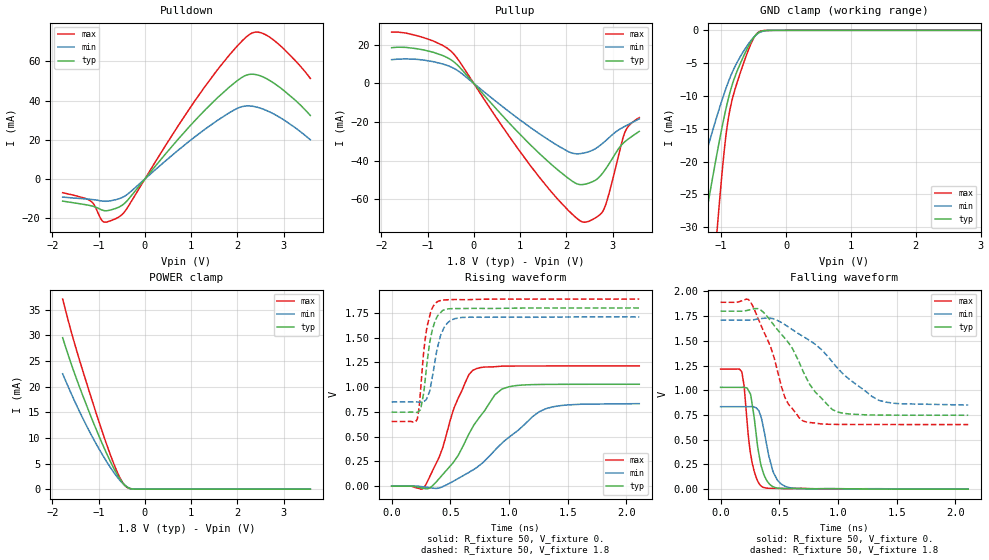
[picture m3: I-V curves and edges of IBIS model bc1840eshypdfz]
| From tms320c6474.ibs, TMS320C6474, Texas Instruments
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|   MODEL bc1840eshypdfz
[Model] bc1840eshypdfz
Model_type I/O
|C_comp_off 861.284f 847.135f 858.339f
|C_comp_on 527.297f 518.909f 520.66f
C_comp 694.29f 683.022f 689.5f
|Rth_i 17.068Meg 5.207Meg 37.052Meg
|Rth_r 37.693 52.451 28.255
|Rth_f 35.826 49.423 26.843
Vinl = 0.630
Vinh = 1.170
Vmeas = 0.9
Cref = 5pF
[Model Spec]
||   Typ   Min   Max
S_overshoot_high   2.100   2.010   2.190
Vinh   1.170   1.111   1.229
Vmeas   0.900   0.855   0.945
Vinl   0.630   0.599   0.662
S_overshoot_low   -0.300  -0.300  -0.300
[Receiver Thresholds]
Vth   = 0.900V
Vth_min = 0.855V
Vth_max = 0.945V
Vinh_ac = +270mV   || Undefined so set to Vinh_dc level
Vinh_dc = +270mV
Vinl_dc = -270mV
Vinl_ac = -270mV   || Undefined so set to Vinl_dc level
Tslew_ac = 5.0ns   || Undefined in specification - set to large value
|| Pointer to HSPICE models:
|ff ti_bc1840eshypdfz.mod ti_bc1840eshypdfz_ff
|tt ti_bc1840eshypdfz.mod ti_bc1840eshypdfz_tt
|ss ti_bc1840eshypdfz.mod ti_bc1840eshypdfz_ss
|| Spice2IBIS controls:
|View_IV No
[Temperature Range]  25   105   -40
|corevdd   1.100  1.045  1.155
[Voltage Range]   1.8   1.71   1.89
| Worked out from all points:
|   slope of the pulldown table from 0 to 0.27 V, typ, clamps not added: 34.7 ohm
|   slope of the pullup table from 0 to 0.27 V, typ, clamps not added: 36.5 ohm
|   GND clamp passes 1 mA (typ) near -0.49 V on its own axis
|   POWER clamp passes 1 mA (typ) near -0.46 V on its own axis
|   rising waveform, R_fixture 50, V_fixture 0.: 20-80 % time 324ps typ, 473ps min, 216ps max; typ from 0 V to 1.03 V
|   rising waveform, R_fixture 50, V_fixture 1.8: 20-80 % time 74.1ps typ, 88.5ps min, 65.9ps max; typ from 0.747 V to 1.8 V
|   falling waveform, R_fixture 50, V_fixture 0.: 20-80 % time 79.8ps typ, 93.5ps min, 67.9ps max; typ from 1.03 V to 0 V
|   falling waveform, R_fixture 50, V_fixture 1.8: 20-80 % time 326ps typ, 487ps min, 211ps max; typ from 1.8 V to 0.748 V
[Pulldown]
-1.779V   -11.3mA    -9.255mA   -7.029mA
-1.172V   -13.64mA   -10.42mA   -11.28mA
-885.2mV  -16.14mA   -11.37mA   -21.98mA
-500.8mV  -13.54mA   -9.552mA   -18.3mA
712mV     20.11mA    14.53mA    26.88mA
1.308V    35.38mA    25.54mA    47.47mA
1.973V    49.72mA    35.76mA    67.24mA
2.309V    53.44mA    37.14mA    74.38mA
2.531V    52.27mA    35.84mA    74.42mA
2.807V    48.57mA    32.88mA    70.44mA
3.257V    40.06mA    26.03mA    60.25mA
3.576V    32.4mA     20.01mA    51.29mA
[Pullup]
-1.776V   18.46mA    12.27mA    26.51mA
-1.094V   17.34mA    12.09mA    23.74mA
-449.6mV  11.48mA    8.028mA    15.63mA
1.218V    -31.64mA   -22.7mA    -42.35mA
2.035V    -48.96mA   -35.19mA   -65.49mA
2.339V    -52.35mA   -36.21mA   -71.56mA
2.62V     -50.22mA   -33.91mA   -69.7mA
2.799V    -46.01mA   -30.75mA   -65.79mA
2.907V    -42.28mA   -28.47mA   -58.43mA
3.264V    -30.24mA   -22.25mA   -25.49mA
3.384V    -28.03mA   -20.76mA   -21.13mA
3.579V    -24.83mA   -18.32mA   -17.71mA
[GND Clamp]
-1.779V   -59.56mA   -37.99mA   -119.5mA
-1.529V   -45.23mA   -29.11mA   -89.37mA
-1.387V   -37mA      -24.1mA    -71.41mA
-1.191V   -25.75mA   -17.29mA   -46.39mA
-1.053V   -18.18mA   -12.7mA    -29.3mA
-937.4mV  -12.45mA   -9.168mA   -16.96mA
-897.4mV  -10.73mA   -8.067mA   -13.92mA
-848.4mV  -8.901mA   -6.841mA   -11.32mA
-581.4mV  -2.472mA   -2.093mA   -3.018mA
-492.4mV  -1.021mA   -996.9uA   -1.09mA
-412.3mV  -275.8uA   -354.1uA   -211.8uA
3.576V    0A         0A         0A
[Power Clamp]
-1.779V   29.56mA    22.51mA    37.1mA
-1.614V   24.99mA    19.08mA    31.43mA
-1.455V   20.94mA    15.94mA    26.43mA
-1.164V   14.12mA    10.66mA    17.94mA
-930.5mV  9.056mA    6.904mA    11.45mA
-739.7mV  5.286mA    4.151mA    6.541mA
-601.9mV  2.905mA    2.406mA    3.416mA
-490.6mV  1.362mA    1.232mA    1.427mA
-400.5mV  513.7uA    525.3uA    451uA
-321mV    131.2uA    160.6uA    101.3uA
-225.5mV  9.942uA    19.46uA    5.634uA
3.579V    0A         0A         0A
[Ramp]
dV/dt_r .618/324.071p .501/473.431p .729/215.934p
dV/dt_f .632/326.322p .516/488.075p .742/210.701p
[Rising Waveform]
R_fixture = 50
V_fixture = 0.
0s        0V         1.05uV     0V
270ps     -21.74mV   -7.257mV   -23.39mV
325ps     -19.33mV   -14.8mV    96.12mV
405ps     75.94mV    -17.84mV   293.2mV
525ps     238.2mV    48.99mV    764.2mV
655ps     518.9mV    136.6mV    1.118V
720ps     649.3mV    183.5mV    1.186V
940ps     980.6mV    433.6mV    1.212V
1.32ns    1.028V     784.7mV    1.214V
2.11ns    1.029V     833.3mV    1.214V
[Rising Waveform]
R_fixture = 50
V_fixture = 1.8
V_fixture_min = 1.71
V_fixture_max = 1.89
0s        747.2mV    850.2mV    653.1mV
215ps     744.7mV    850.2mV    669.4mV
235ps     760.4mV    849.5mV    797.8mV
250ps     791.7mV    849.9mV    1.019V
300ps     1.23V      887.2mV    1.597V
345ps     1.57V      1.092V     1.795V
400ps     1.731V     1.443V     1.869V
475ps     1.789V     1.648V     1.883V
595ps     1.794V     1.704V     1.884V
2.11ns    1.8V       1.71V      1.89V
[Falling Waveform]
R_fixture = 50
V_fixture = 0.
0s        1.03V      834.2mV    1.215V
180ps     1.03V      834.2mV    1.187V
200ps     1.03V      834.2mV    1.047V
230ps     1.015V     834.2mV    626mV
270ps     852.2mV    834.1mV    260.6mV
320ps     399mV      801mV      73.28mV
365ps     162.1mV    622.5mV    17.59mV
450ps     23.32mV    168.4mV    8.658mV
580ps     6.889mV    17.31mV    5.07mV
2.11ns    375.6uV    685.6uV    140.3uV
[Falling Waveform]
R_fixture = 50
V_fixture = 1.8
V_fixture_min = 1.71
V_fixture_max = 1.89
0s        1.8V       1.71V      1.89V
255ps     1.816V     1.71V      1.893V
340ps     1.813V     1.724V     1.668V
430ps     1.697V     1.728V     1.426V
550ps     1.522V     1.662V     922.7mV
700ps     1.2V       1.546V     691.5mV
805ps     985.3mV    1.467V     669.1mV
950ps     807.3mV    1.29V      655.7mV
1.35ns    749.4mV    897.8mV    653.8mV
2.11ns    747.6mV    851.1mV    653.4mV
